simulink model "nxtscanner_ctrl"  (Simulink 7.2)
settings: Solver=FixedStepDiscrete  SolverMode=SingleTasking  StartTime=0  StopTime=inf  FixedStep=0.001  RelTol=1e-3
PreLoadFcn:
  | mode_control_prm;
  | scanner_head_prm;
  | xlsreadsdo('nxtscanner.xls','mpt');
undefined symbols (not defined in the file or in its folder): ScannerBufferInfoEnum
libraries: ecrobot_nxt_lib x31, nxtscanner_lib x4, PolySpaceLibForEmbeddedCoder x1

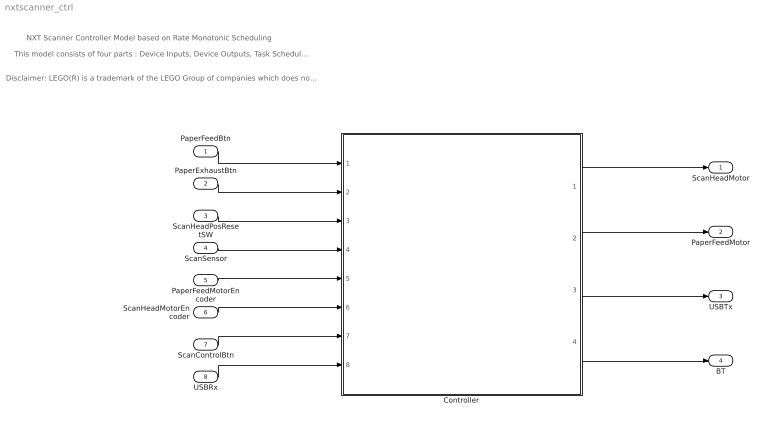
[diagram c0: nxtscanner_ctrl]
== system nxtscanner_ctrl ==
  note: Disclaimer: LEGO(R) is a trademark of the LEGO Group of companies which does not sponsor, authorize or endorse this demo. LEGO(R) and Mindstorms(R) are registered trademarks of The LEGO Group.
  note: NXT Scanner Controller Model based on Rate Monotonic Scheduling
  note: This model consists of four parts : Device Inputs, Device Outputs, Task Scheduler, and Application Task Subsystems.
  PaperFeedBtn : Inport  OutDataType=sfix(16)  OutScaling=2^0
  PaperExhaustBtn : Inport  Port=2  OutDataType=sfix(16)  OutScaling=2^0
  ScanHeadPosResetSW : Inport  Port=3  OutDataType=sfix(16)  OutScaling=2^0
  ScanSensor : Inport  Port=4  OutDataType=sfix(16)  OutScaling=2^0
  PaperFeedMotorEncoder : Inport  Port=5  OutDataType=sfix(16)  OutScaling=2^0
  ScanHeadMotorEncoder : Inport  Port=6  OutDataType=sfix(16)  OutScaling=2^0
  ScanControlBtn : Inport  Port=7  OutDataType=sfix(16)  OutScaling=2^0
  USBRx : Inport  Port=8  OutDataType=sfix(16)  OutScaling=2^0
  Controller : Subsystem
  ScanHeadMotor : Outport  OutDataType=sfix(16)  OutScaling=2^0
  PaperFeedMotor : Outport  Port=2  OutDataType=sfix(16)  OutScaling=2^0
  USBTx : Outport  Port=3  OutDataType=sfix(16)  OutScaling=2^0
  BT : Outport  Port=4  OutDataType=sfix(16)  OutScaling=2^0
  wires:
  Controller/1(ScanHeadMotor) -> ScanHeadMotor/1
  Controller/2(PaperFeedMotor) -> PaperFeedMotor/1
  Controller/3(USBTx) -> USBTx/1
  PaperFeedBtn/1 -> Controller/1(PaperFeedBtn)
  PaperExhaustBtn/1 -> Controller/2(PaperExhaustBtn)
  ScanHeadPosResetSW/1 -> Controller/3(ScanHeadPosResetSW)
  ScanSensor/1 -> Controller/4(ScanSensor)
  PaperFeedMotorEncoder/1 -> Controller/5(PaperFeedMotorEncoder)
  ScanHeadMotorEncoder/1 -> Controller/6(ScanHeadMotorEncoder)
  ScanControlBtn/1 -> Controller/7(ScanControlBtn)
  USBRx/1 -> Controller/8(USBRx)
  Controller/4(BT) -> BT/1

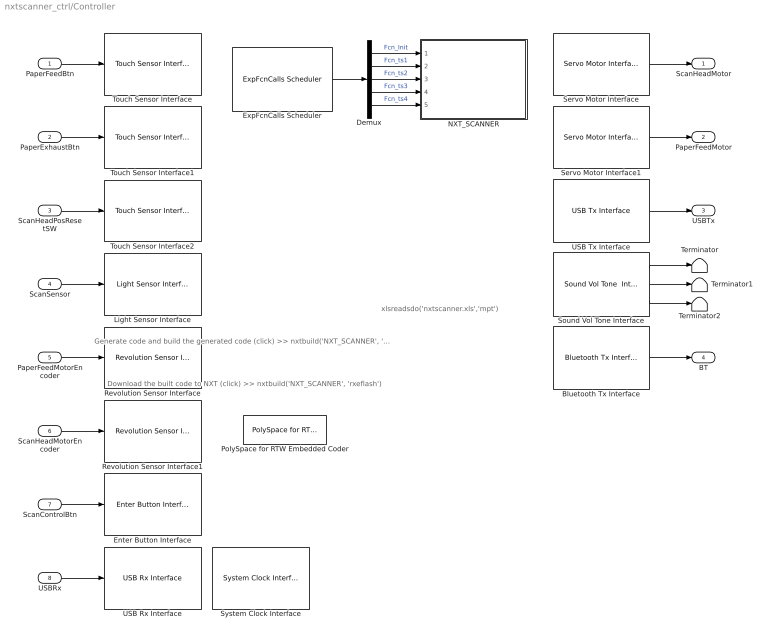
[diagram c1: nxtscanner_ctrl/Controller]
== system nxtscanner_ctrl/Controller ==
  note: Generate code and build the generated code (click) >> nxtbuild('NXT_SCANNER', 'build')
  note: Download the built code to NXT (click) >> nxtbuild('NXT_SCANNER', 'rxeflash')
  note: xlsreadsdo('nxtscanner.xls','mpt')
  PaperFeedBtn : Inport
  PaperExhaustBtn : Inport  Port=2
  ScanHeadPosResetSW : Inport  Port=3
  ScanSensor : Inport  Port=4
  PaperFeedMotorEncoder : Inport  Port=5
  ScanHeadMotorEncoder : Inport  Port=6
  ScanControlBtn : Inport  Port=7
  USBRx : Inport  Port=8
  Bluetooth Tx Interface : ecrobot_nxt_lib/Bluetooth Tx Interface  SystemSampleTime=-1
  Demux : Demux  Outputs=5
  Enter Button Interface : ecrobot_nxt_lib/Enter Button Interface  Priority=-1  SystemSampleTime=-1
  ExpFcnCalls Scheduler : ecrobot_nxt_lib/ExpFcnCalls Scheduler  Priority=0  fcname='Fcn_Init', 'Fcn_ts1', 'Fcn_ts2', 'Fcn_ts3', 'Fcn_ts4'  fctrigger=[0 2 10 20 60]  ts=0.001  platform=JSP  stacksize=[512 512 512 512 512]  bd_mode=Slave
  Light Sensor Interface : ecrobot_nxt_lib/Light Sensor Interface  Priority=-1  SystemSampleTime=-1  ip=S4
  NXT_SCANNER : Subsystem
  PolySpace for RTW Embedded Coder : PolySpaceLibForEmbeddedCoder/PolySpace for RTW Embedded Coder  Description=PolySpace for RTW\nEmbedded Coder  SystemSampleTime=-1
  Revolution Sensor Interface : ecrobot_nxt_lib/Revolution Sensor Interface  Priority=-1  SystemSampleTime=-1  ip=B
  Revolution Sensor Interface1 : ecrobot_nxt_lib/Revolution Sensor Interface  Priority=-1  SystemSampleTime=-1  ip=C
  Servo Motor Interface : ecrobot_nxt_lib/Servo Motor Interface  Priority=1  SystemSampleTime=-1  ip=B  mode=Brake
  Servo Motor Interface1 : ecrobot_nxt_lib/Servo Motor Interface  Priority=1  SystemSampleTime=-1  ip=C  mode=Brake
  Sound Vol Tone Interface : ecrobot_nxt_lib/Sound Vol Tone  Interface  Priority=1  SystemSampleTime=-1
  System Clock Interface : ecrobot_nxt_lib/System Clock Interface  Priority=-1  SystemSampleTime=-1
  Terminator : Terminator
  Terminator1 : Terminator
  Terminator2 : Terminator
  Touch Sensor Interface : ecrobot_nxt_lib/Touch Sensor Interface  Priority=-1  SystemSampleTime=-1  ip=S1
  Touch Sensor Interface1 : ecrobot_nxt_lib/Touch Sensor Interface  Priority=-1  SystemSampleTime=-1  ip=S2
  Touch Sensor Interface2 : ecrobot_nxt_lib/Touch Sensor Interface  Priority=-1  SystemSampleTime=-1  ip=S3
  USB Rx Interface : ecrobot_nxt_lib/USB Rx Interface  Priority=-1  SystemSampleTime=-1
  USB Tx Interface : ecrobot_nxt_lib/USB Tx Interface  Priority=1  SystemSampleTime=-1
  ScanHeadMotor : Outport
  PaperFeedMotor : Outport  Port=2
  USBTx : Outport  Port=3
  BT : Outport  Port=4
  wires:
  ExpFcnCalls Scheduler/1 -> Demux/1
  Demux/1 -> NXT_SCANNER/1(In1)  "Fcn_Init"
  Demux/2 -> NXT_SCANNER/2(In2)  "Fcn_ts1"
  Demux/3 -> NXT_SCANNER/3(In3)  "Fcn_ts2"
  Servo Motor Interface/1 -> ScanHeadMotor/1
  PaperFeedBtn/1 -> Touch Sensor Interface/1
  Servo Motor Interface1/1 -> PaperFeedMotor/1
  PaperExhaustBtn/1 -> Touch Sensor Interface1/1
  ScanHeadPosResetSW/1 -> Touch Sensor Interface2/1
  USB Tx Interface/1 -> USBTx/1
  ScanSensor/1 -> Light Sensor Interface/1
  PaperFeedMotorEncoder/1 -> Revolution Sensor Interface/1
  ScanHeadMotorEncoder/1 -> Revolution Sensor Interface1/1
  ScanControlBtn/1 -> Enter Button Interface/1
  USBRx/1 -> USB Rx Interface/1
  Sound Vol Tone Interface/1 -> Terminator/1
  Sound Vol Tone Interface/2 -> Terminator1/1
  Sound Vol Tone Interface/3 -> Terminator2/1
  Bluetooth Tx Interface/1 -> BT/1
  Demux/4 -> NXT_SCANNER/4(In4)  "Fcn_ts3"
  Demux/5 -> NXT_SCANNER/5(In5)  "Fcn_ts4"

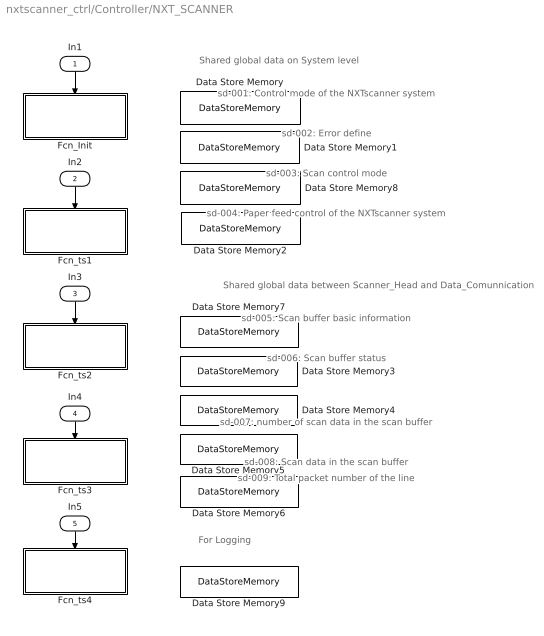
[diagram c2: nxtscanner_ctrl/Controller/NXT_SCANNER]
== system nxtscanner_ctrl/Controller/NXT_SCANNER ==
  note: Shared global data on System level
  note: Shared global data between Scanner_Head and Data_Comunnication
  note: sd-001: Control mode of the NXTscanner system
  note: sd-002: Error define
  note: sd-003: Scan control mode
  note: sd-004: Paper feed control of the NXTscanner system
  note: sd-005: Scan buffer basic information
  note: sd-006: Scan buffer status
  note: sd-007: number of scan data in the scan buffer
  note: sd-008: Scan data in the scan buffer
  note: sd-009: Total packet number of the line
  note: For Logging
  In1 : Inport  Orientation=down
  In2 : Inport  Orientation=down  Port=2
  In3 : Inport  Orientation=down  Port=3
  In4 : Inport  Orientation=down  Port=4
  In5 : Inport  Orientation=down  Port=5
  Data Store Memory : DataStoreMemory  DataStoreName=ControlMode  ReadBeforeWriteMsg=warning  WriteAfterWriteMsg=warning  WriteAfterReadMsg=warning  InitialValue=ControlModeEnum.INITIALIZE  DataType=Specify via dialog  OutDataType=Enum: ControlModeEnum  OutDataTypeStr=Enum: ControlModeEnum
  Data Store Memory1 : DataStoreMemory  DataStoreName=ErrorCode  ReadBeforeWriteMsg=warning  WriteAfterWriteMsg=warning  WriteAfterReadMsg=warning  InitialValue=ErrorCodeEnum.NO_ERROR  DataType=Specify via dialog  OutDataType=Enum: ErrorCodeEnum  OutDataTypeStr=Enum: ErrorCodeEnum
  Data Store Memory2 : DataStoreMemory  DataStoreName=FeedMode  ReadBeforeWriteMsg=warning  WriteAfterWriteMsg=warning  WriteAfterReadMsg=warning  InitialValue=FeedModeEnum.FEED_INIT  DataType=Specify via dialog  OutDataType=Enum: FeedModeEnum  OutDataTypeStr=Enum: FeedModeEnum
  Data Store Memory3 : DataStoreMemory  DataStoreName=ScannerBuffer_Status  ReadBeforeWriteMsg=warning  WriteAfterWriteMsg=warning  WriteAfterReadMsg=warning  InitialValue=[0;0]  DataType=uint16  OutDataType=Enum: ScannerBufferStatusEnum  OutDataTypeStr=uint16
  Data Store Memory4 : DataStoreMemory  DataStoreName=ScannerBuffer_Number  ReadBeforeWriteMsg=warning  WriteAfterWriteMsg=warning  WriteAfterReadMsg=warning  InitialValue=[0;0]  DataType=uint8  OutDataType=Enum: FeedModeEnum  OutDataTypeStr=uint8
  Data Store Memory5 : DataStoreMemory  DataStoreName=ScannerBuffer_Data  ReadBeforeWriteMsg=warning  WriteAfterWriteMsg=warning  WriteAfterReadMsg=warning  InitialValue=[0 0 0 0 0 0 0 0 0 0 0 0 0 0 0 0 0 0 0 0 0 0 0 0 0 0 0 0 0 0; 0 0 0 0 0 0 0 0 0 0 0 0 0 0 0 0 0 0 0 0 0 0 0 0 0 0 0 0 0 0]  DataType=uint16  OutDataType=Enum: FeedModeEnum  OutDataTypeStr=uint16
  Data Store Memory6 : DataStoreMemory  DataStoreName=ScannerBuffer_Pnum  ReadBeforeWriteMsg=warning  WriteAfterWriteMsg=warning  WriteAfterReadMsg=warning  InitialValue=[0;0]  DataType=uint8  OutDataType=Enum: FeedModeEnum  OutDataTypeStr=uint8
  Data Store Memory7 : DataStoreMemory  DataStoreName=ScannerBuffer_Info  ReadBeforeWriteMsg=warning  WriteAfterWriteMsg=warning  WriteAfterReadMsg=warning  InitialValue=[ScannerBufferInfoEnum.TRANS_FINISH;ScannerBufferInfoEnum.TRANS_FINISH]  DataType=Specify via dialog  OutDataType=Enum: ScannerBufferInfoEnum  OutDataTypeStr=Enum: ScannerBufferInfoEnum
  Data Store Memory8 : DataStoreMemory  DataStoreName=ScanMode  ReadBeforeWriteMsg=warning  WriteAfterWriteMsg=warning  WriteAfterReadMsg=warning  InitialValue=ScanModeEnum.SCAN_INIT  DataType=Specify via dialog  OutDataType=Enum: ScanModeEnum  OutDataTypeStr=Enum: ScanModeEnum
  Data Store Memory9 : DataStoreMemory  DataStoreName=paper_feed_pwm  ReadBeforeWriteMsg=warning  WriteAfterWriteMsg=warning  WriteAfterReadMsg=warning  DataType=int8  OutDataType=Enum: FeedModeEnum  OutDataTypeStr=int8
  Fcn_Init : Subsystem  TreatAsAtomicUnit=on
  Fcn_ts1 : Subsystem  TreatAsAtomicUnit=on
  Fcn_ts2 : Subsystem  TreatAsAtomicUnit=on
  Fcn_ts3 : Subsystem  TreatAsAtomicUnit=on
  Fcn_ts4 : Subsystem  TreatAsAtomicUnit=on
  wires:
  In1/1 -> Fcn_Init/Trigger
  In2/1 -> Fcn_ts1/Trigger
  In3/1 -> Fcn_ts2/Trigger
  In5/1 -> Fcn_ts4/Trigger
  In4/1 -> Fcn_ts3/Trigger

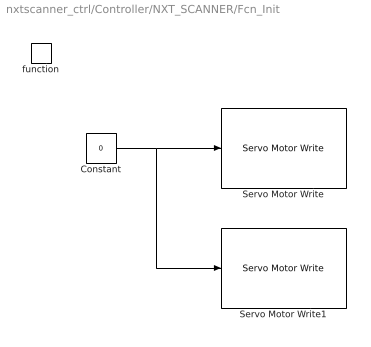
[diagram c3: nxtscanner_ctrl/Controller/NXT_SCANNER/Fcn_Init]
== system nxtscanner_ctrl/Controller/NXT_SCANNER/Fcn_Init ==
  function : TriggerPort  TriggerType=function-call
  Constant : Constant  Value=0  OutDataType=sfix(16)  OutScaling=2^0  OutDataTypeStr=Inherit: Inherit via back propagation
  Servo Motor Write : ecrobot_nxt_lib/Servo Motor Write  SystemSampleTime=-1  ip=B
  Servo Motor Write1 : ecrobot_nxt_lib/Servo Motor Write  SystemSampleTime=-1  ip=C
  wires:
  Constant/1 -> Servo Motor Write/1, Servo Motor Write1/1

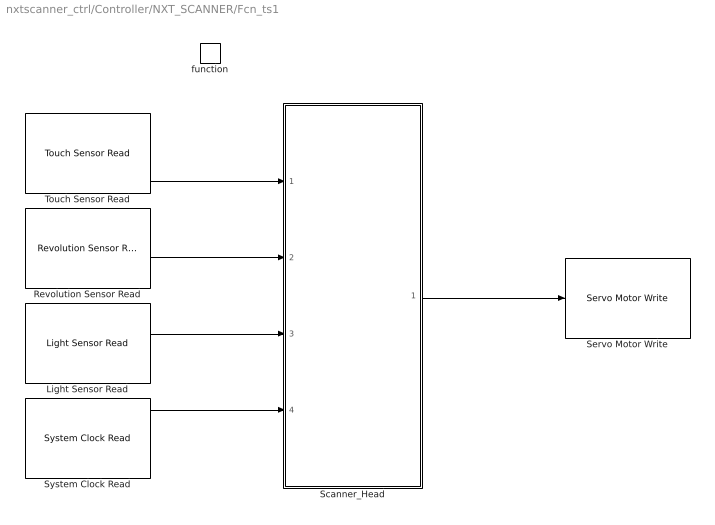
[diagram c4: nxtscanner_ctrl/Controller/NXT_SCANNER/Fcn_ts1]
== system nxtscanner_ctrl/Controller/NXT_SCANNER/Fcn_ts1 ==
  function : TriggerPort  TriggerType=function-call
  Light Sensor Read : ecrobot_nxt_lib/Light Sensor Read  SystemSampleTime=-1  ip=S4
  Revolution Sensor Read : ecrobot_nxt_lib/Revolution Sensor Read  SystemSampleTime=-1  ip=C
  Scanner_Head : Subsystem
  Servo Motor Write : ecrobot_nxt_lib/Servo Motor Write  SystemSampleTime=-1  ip=C
  System Clock Read : ecrobot_nxt_lib/System Clock Read  SystemSampleTime=-1
  Touch Sensor Read : ecrobot_nxt_lib/Touch Sensor Read  SystemSampleTime=-1  ip=S3
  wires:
  Revolution Sensor Read/1 -> Scanner_Head/2(Encoder)
  Touch Sensor Read/1 -> Scanner_Head/1(Touch)
  Light Sensor Read/1 -> Scanner_Head/3(LightSensor)
  Scanner_Head/1(PWM) -> Servo Motor Write/1
  System Clock Read/1 -> Scanner_Head/4(SystemClock)

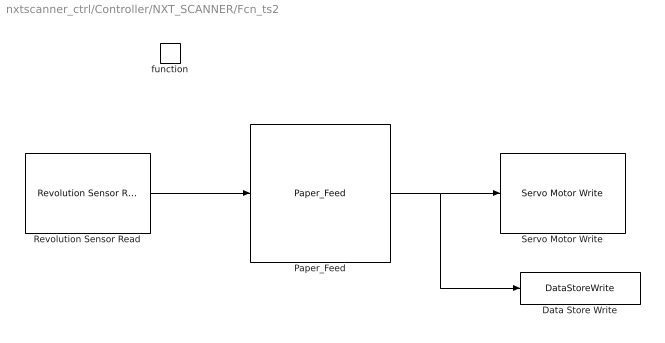
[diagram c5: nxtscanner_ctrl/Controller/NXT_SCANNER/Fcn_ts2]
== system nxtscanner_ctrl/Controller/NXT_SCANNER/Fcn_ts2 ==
  function : TriggerPort  TriggerType=function-call
  Data Store Write : DataStoreWrite  DataStoreName=paper_feed_pwm  SampleTime=-1
  Paper_Feed : nxtscanner_lib/Paper_Feed  Priority=1  SystemSampleTime=-1
  Revolution Sensor Read : ecrobot_nxt_lib/Revolution Sensor Read  SystemSampleTime=-1  ip=B
  Servo Motor Write : ecrobot_nxt_lib/Servo Motor Write  SystemSampleTime=-1  ip=B
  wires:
  Revolution Sensor Read/1 -> Paper_Feed/1
  Paper_Feed/1 -> Servo Motor Write/1, Data Store Write/1

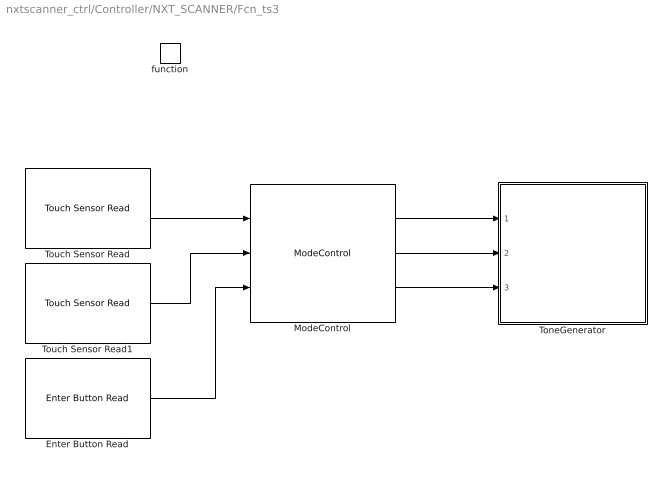
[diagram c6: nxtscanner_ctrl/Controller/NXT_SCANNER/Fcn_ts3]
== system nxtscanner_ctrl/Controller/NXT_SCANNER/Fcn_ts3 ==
  function : TriggerPort  TriggerType=function-call
  Enter Button Read : ecrobot_nxt_lib/Enter Button Read  SystemSampleTime=-1
  ModeControl : nxtscanner_lib/ModeControl  Priority=-1  SystemSampleTime=-1
  ToneGenerator : Subsystem
  Touch Sensor Read : ecrobot_nxt_lib/Touch Sensor Read  SystemSampleTime=-1  ip=S1
  Touch Sensor Read1 : ecrobot_nxt_lib/Touch Sensor Read  SystemSampleTime=-1  ip=S2
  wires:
  ModeControl/3 -> ToneGenerator/3(Vol)
  ModeControl/2 -> ToneGenerator/2(Dur)
  ModeControl/1 -> ToneGenerator/1(Freq)
  Enter Button Read/1 -> ModeControl/3
  Touch Sensor Read1/1 -> ModeControl/2
  Touch Sensor Read/1 -> ModeControl/1

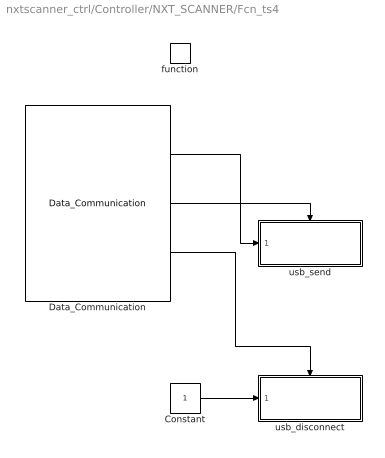
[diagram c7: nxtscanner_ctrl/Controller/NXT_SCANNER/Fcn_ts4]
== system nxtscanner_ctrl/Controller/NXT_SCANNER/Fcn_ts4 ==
  function : TriggerPort  TriggerType=function-call
  Constant : Constant  OutDataType=sfix(16)  OutScaling=2^0  OutDataTypeStr=Inherit: Inherit via back propagation  SampleTime=-1
  Data_Communication : nxtscanner_lib/Data_Communication  SystemSampleTime=-1
  usb_disconnect : Subsystem  TreatAsAtomicUnit=on
  usb_send : Subsystem  TreatAsAtomicUnit=on
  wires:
  Data_Communication/2 -> usb_send/Trigger
  Data_Communication/1 -> usb_send/1(In1)
  Data_Communication/3 -> usb_disconnect/Trigger
  Constant/1 -> usb_disconnect/1(In1)

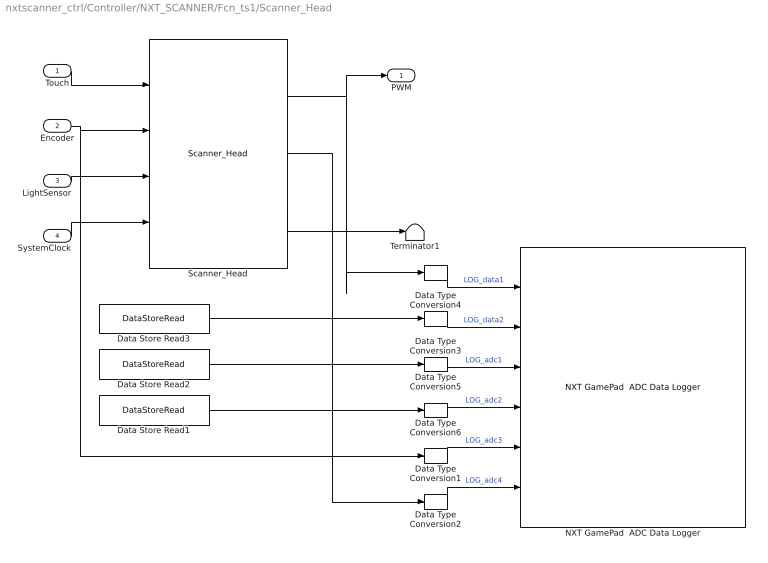
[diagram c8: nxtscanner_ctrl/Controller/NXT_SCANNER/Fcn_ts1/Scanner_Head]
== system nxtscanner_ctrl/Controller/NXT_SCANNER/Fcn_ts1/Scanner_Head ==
  Touch : Inport
  Encoder : Inport  Port=2
  LightSensor : Inport  Port=3
  SystemClock : Inport  Port=4
  Data Store Read1 : DataStoreRead  DataStoreName=ScanMode  SampleTime=-1
  Data Store Read2 : DataStoreRead  DataStoreName=ControlMode  SampleTime=-1
  Data Store Read3 : DataStoreRead  DataStoreName=paper_feed_pwm  SampleTime=-1
  Data Type Conversion{1..6} (6 alike) : DataTypeConversion  OutDataType=sfix(16)  OutScaling=2^0
  NXT GamePad  ADC Data Logger : ecrobot_nxt_lib/NXT GamePad  ADC Data Logger
  Scanner_Head : nxtscanner_lib/Scanner_Head  SystemSampleTime=-1
  Terminator1 : Terminator
  PWM : Outport
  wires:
  Touch/1 -> Scanner_Head/1
  Encoder/1 -> Scanner_Head/2, Data Type Conversion1/1
  Scanner_Head/1 -> PWM/1, Data Type Conversion4/1
  Data Type Conversion4/1 -> NXT GamePad  ADC Data Logger/1  "LOG_data1"
  Data Type Conversion1/1 -> NXT GamePad  ADC Data Logger/5  "LOG_adc3"
  Data Type Conversion2/1 -> NXT GamePad  ADC Data Logger/6  "LOG_adc4"
  Data Store Read1/1 -> Data Type Conversion6/1
  Data Type Conversion6/1 -> NXT GamePad  ADC Data Logger/4  "LOG_adc2"
  Data Store Read2/1 -> Data Type Conversion5/1
  Data Type Conversion5/1 -> NXT GamePad  ADC Data Logger/3  "LOG_adc1"
  SystemClock/1 -> Scanner_Head/4
  LightSensor/1 -> Scanner_Head/3
  Data Store Read3/1 -> Data Type Conversion3/1
  Data Type Conversion3/1 -> NXT GamePad  ADC Data Logger/2  "LOG_data2"
  Scanner_Head/2 -> Data Type Conversion2/1
  Scanner_Head/3 -> Terminator1/1

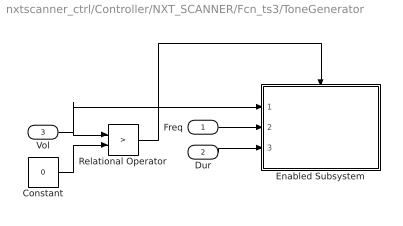
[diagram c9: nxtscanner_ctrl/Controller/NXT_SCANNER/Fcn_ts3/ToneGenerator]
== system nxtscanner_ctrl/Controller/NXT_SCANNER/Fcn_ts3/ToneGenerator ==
  Freq : Inport
  Dur : Inport  Port=2
  Vol : Inport  Port=3
  Constant : Constant  Value=0  OutDataTypeMode=uint32  OutDataType=sfix(16)  OutScaling=2^0  OutDataTypeStr=uint32
  Enabled Subsystem : Subsystem  TreatAsAtomicUnit=on
  Relational Operator : RelationalOperator  Operator=>  LogicOutDataTypeMode=boolean  OutDataTypeStr=boolean
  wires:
  Dur/1 -> Enabled Subsystem/3(Dur)
  Freq/1 -> Enabled Subsystem/2(Freq)
  Relational Operator/1 -> Enabled Subsystem/Trigger
  Constant/1 -> Relational Operator/2
  Vol/1 -> Relational Operator/1, Enabled Subsystem/1(Vol)

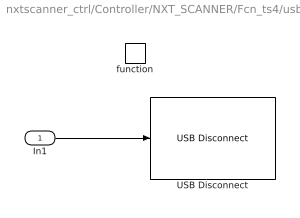
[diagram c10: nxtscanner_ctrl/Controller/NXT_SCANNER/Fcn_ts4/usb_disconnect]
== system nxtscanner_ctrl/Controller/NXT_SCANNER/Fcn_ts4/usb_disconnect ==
  In1 : Inport  OutDataType=sfix(16)  OutScaling=2^0
  function : TriggerPort  TriggerType=function-call
  USB Disconnect : ecrobot_nxt_lib/USB Disconnect
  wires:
  In1/1 -> USB Disconnect/1

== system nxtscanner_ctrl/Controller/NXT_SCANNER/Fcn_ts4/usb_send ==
  In1 : Inport  OutDataType=sfix(16)  OutScaling=2^0
  function : TriggerPort  TriggerType=function-call
  USB Tx Write : ecrobot_nxt_lib/USB Tx Write
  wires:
  In1/1 -> USB Tx Write/1

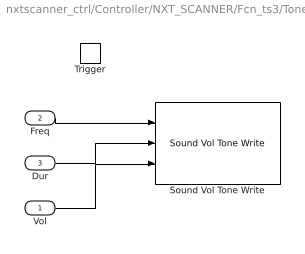
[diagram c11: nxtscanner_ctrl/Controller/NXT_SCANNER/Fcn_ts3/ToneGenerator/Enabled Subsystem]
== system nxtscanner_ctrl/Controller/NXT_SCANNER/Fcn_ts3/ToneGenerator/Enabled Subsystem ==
  Vol : Inport  OutDataType=sfix(16)  OutScaling=2^0
  Freq : Inport  Port=2  OutDataType=sfix(16)  OutScaling=2^0
  Dur : Inport  Port=3  OutDataType=sfix(16)  OutScaling=2^0
  Trigger : TriggerPort
  Sound Vol Tone Write : ecrobot_nxt_lib/Sound Vol Tone Write
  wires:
  Vol/1 -> Sound Vol Tone Write/3
  Dur/1 -> Sound Vol Tone Write/2
  Freq/1 -> Sound Vol Tone Write/1
